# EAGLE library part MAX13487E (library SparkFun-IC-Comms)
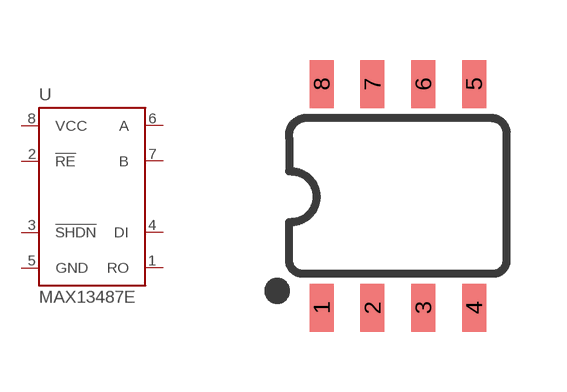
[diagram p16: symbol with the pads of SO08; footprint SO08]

Designator prefix U

## MAX13487E (PROD_ID: IC-13823)  [SO08]
1  RO
2  !RE
3  !SHDN
4  DI
5  GND
6  A
7  B
8  VCC

## Footprint SO08 (pad centres in mm)
SOIC -8 Specifications: Pin count: 8 Width: 0.15" Example device(s): MCP2551
smd 0.6 x 1.2: 1 -1.905,-2.8; 2 -0.635,-2.8; 3 0.635,-2.8; 4 1.905,-2.8; 5 1.905,2.8; 6 0.635,2.8; 7 -0.635,2.8; 8 -1.905,2.8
